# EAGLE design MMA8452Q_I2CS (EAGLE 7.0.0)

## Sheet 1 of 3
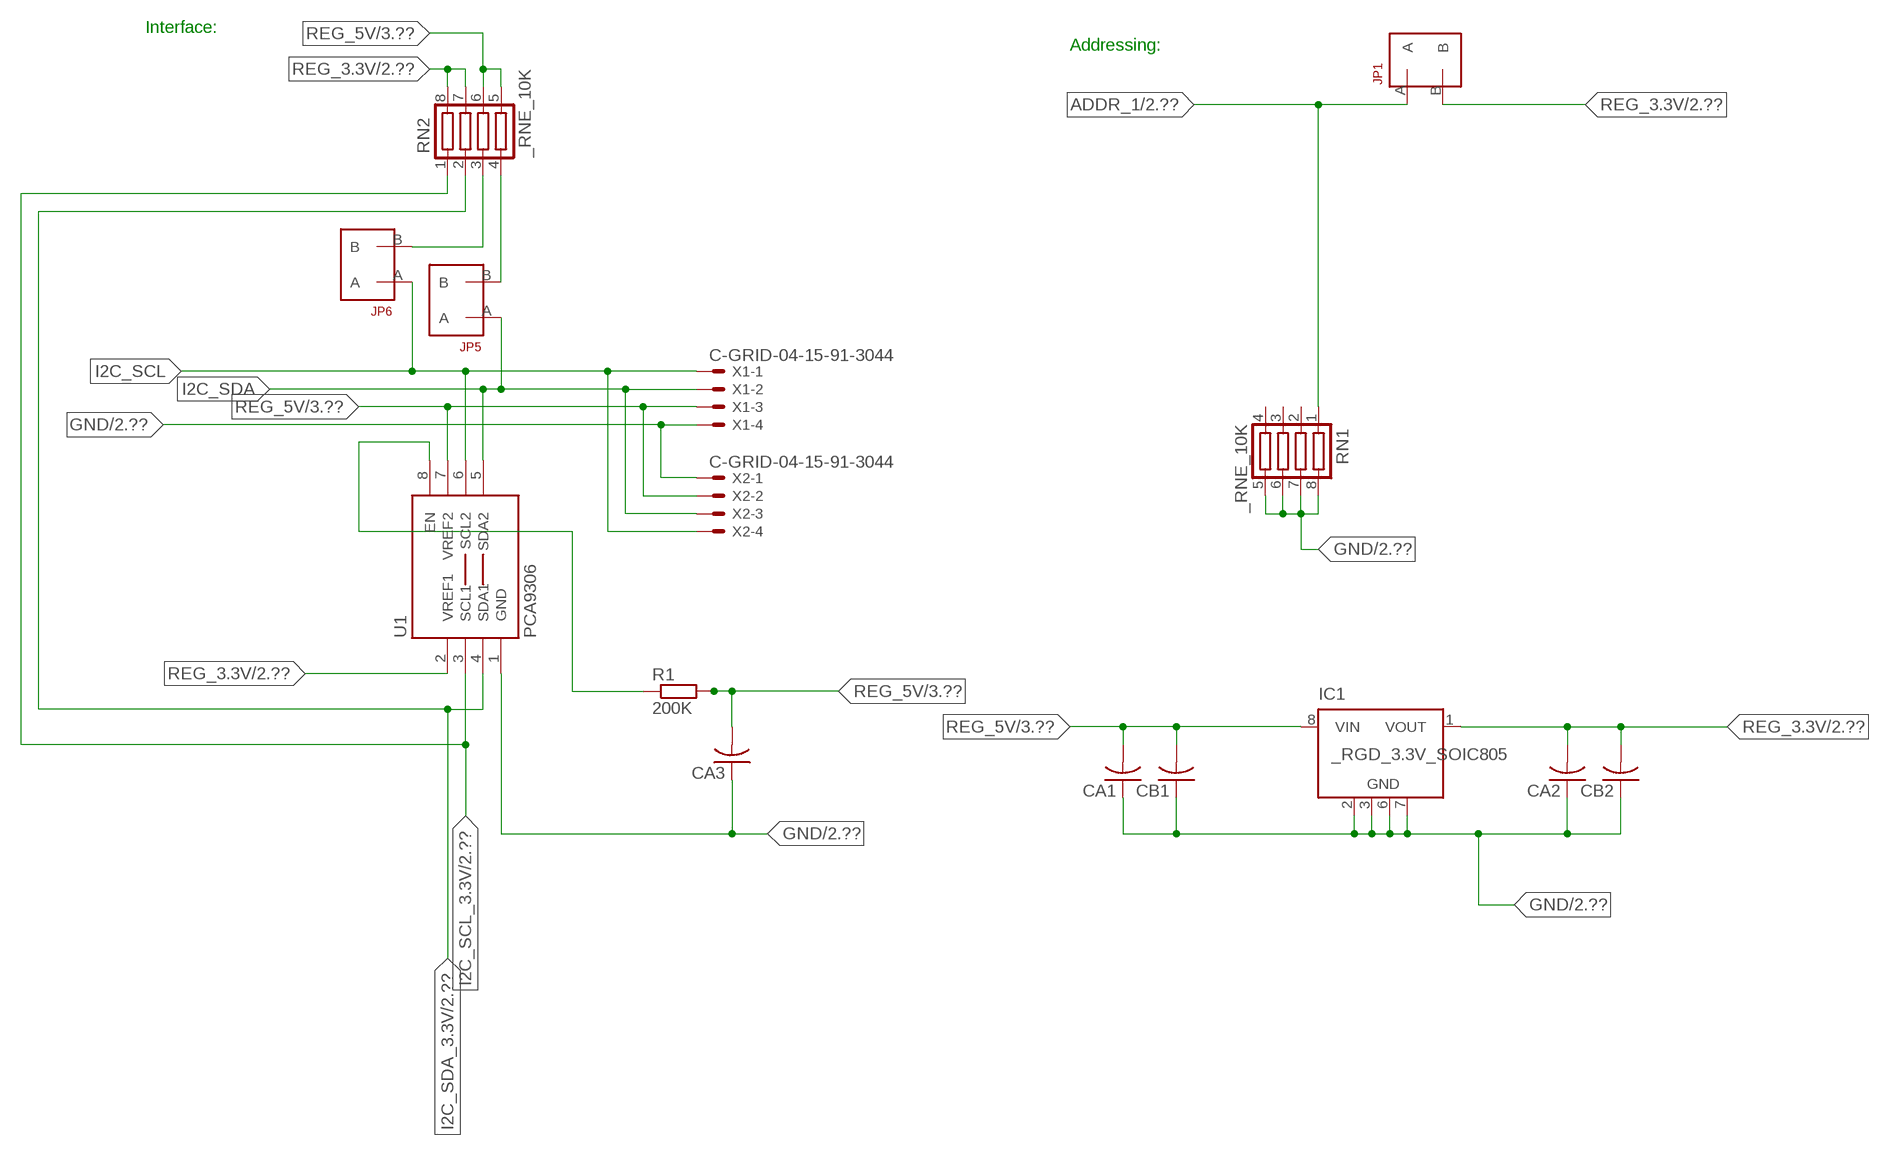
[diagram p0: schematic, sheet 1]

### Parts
CA1  CC1206KRX7R9BB104  [.1UF]
CA2  CC1206KRX7R9BB104  [.1UF]
CA3  CC1206KRX7R9BB104  [.1UF]
CB1  TMK316F106ZL-TC1206K  [TMK316F106ZL-T]
CB2  TMK316F106ZL-TC1206K  [TMK316F106ZL-T]
IC1  _RGD_3.3V_SOIC805  [_RGC_3.3V_SOIC8]
JP1  JUMPER_1X2_2MM  [JUMPER_1X2_2MM]
JP5  JUMPER_1X2_2MM  [JUMPER_1X2_2MM]
JP6  JUMPER_1X2_2MM  [JUMPER_1X2_2MM]
R1  200K  RESISTOR_SMT-0603  [R603]
RN1  _RNE_10K  [RNE]
RN2  _RNE_10K  [RNE]
U1  PCA9306  PCA9306_NCD  [PSOP-8]
X1  C-GRID-04-15-91-3044  [15-91-04]
X2  C-GRID-04-15-91-3044  [15-91-04]

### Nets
ADDR_1: JP1.A RN1.1 ; also sheet 2
GND: CA1.1 CA2.1 CA3.1 CB1.1 CB2.1 IC1.2(GND) IC1.3(GND) IC1.6(GND) IC1.7(GND) RN1.5 RN1.6 RN1.7 RN1.8 U1.1(GND) X1.4 X2.1 ; also sheet 2,3
I2C_SCL: JP6.A U1.6(SCL2) X1.1 X2.4
I2C_SCL_3.3V: RN2.1 U1.3(SCL1) ; also sheet 2
I2C_SDA: JP5.A U1.5(SDA2) X1.2 X2.3
I2C_SDA_3.3V: RN2.2 U1.4(SDA1) ; also sheet 2
N$1: JP6.B RN2.3
N$2: JP5.B RN2.4
N$3: R1.1 U1.8(EN)
REG_3.3V: CA2.2 CB2.2 IC1.1(VOUT) JP1.B RN2.7 RN2.8 U1.2(VREF1) ; also sheet 2
REG_5V: CA1.2 CA3.2 CB1.2 IC1.8(VIN) R1.2 RN2.5 RN2.6 U1.7(VREF2) X1.3 X2.2 ; also sheet 3
Unconnected: IC1.4(NC) IC1.5(NC) RN1.2 RN1.3 RN1.4

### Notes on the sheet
- Interface:
- Addressing:

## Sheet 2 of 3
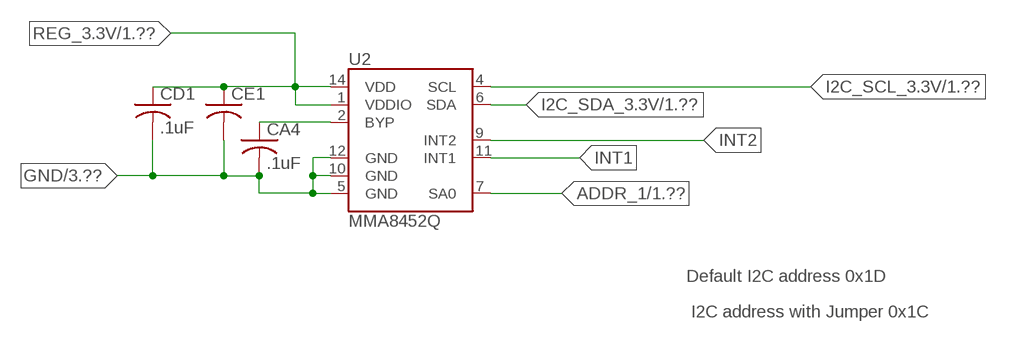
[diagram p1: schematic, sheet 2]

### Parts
CA4  .1uF  CC1206KRX7R9BB104  [.1UF]
CD1  .1uF  CC1206KRX7R9BB103C1206K  [CC1206KRX7R9BB103]
CE1  10uF  CC0603JRNPO8BN1020603  [CC0603JRNPO8BN102]
U2  MMA8452Q  [QFN-16_0.5MM]

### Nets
ADDR_1: U2.7(SA0) ; also sheet 1
GND: CA4.2 CD1.2 CE1.2 U2.5(GND) U2.10(GND) U2.12(GND) ; also sheet 1,3
I2C_SCL_3.3V: U2.4(SCL) ; also sheet 1
I2C_SDA_3.3V: U2.6(SDA) ; also sheet 1
INT1: U2.11(INT1)
INT2: U2.9(INT2)
N$6: CA4.1 U2.2(BYP)
REG_3.3V: CD1.1 CE1.1 U2.1(VDDIO) U2.14(VDD) ; also sheet 1

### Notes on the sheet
- Default I2C address 0x1D
- I2C address with Jumper 0x1C

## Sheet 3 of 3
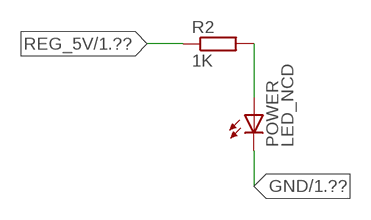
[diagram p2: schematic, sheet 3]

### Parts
POWER  LED_NCD  [CHIPLED_0603]
R2  1K  RESISTOR_SMT-0402  [R402]

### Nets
GND: POWER.C ; also sheet 1,2
N$4: POWER.A R2.2
REG_5V: R2.1 ; also sheet 1

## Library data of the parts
CA1-CA4 = NCD_ULTIMATE_LIBRARY:CC1206KRX7R9BB104: Capacitor CA .1uF 50V SMT C1206K CC1206KRX7R9BB104
CB1 CB2 = NCD_ULTIMATE_LIBRARY:TMK316F106ZL-T: Capacitor CB 10uF SMT 1206 TMK316F106ZL-T
CD1 = NCD_ULTIMATE_LIBRARY:CC1206KRX7R9BB103: Capacitor CD .01uF SMT CC1206KRX7R9BB103 1206
CE1 = NCD_ULTIMATE_LIBRARY:CC0603JRNPO8BN102: Capacitor CE 1uF SMT CC0603JRNPO8BN102 0603
IC1 = NCD_ULTIMATE_LIBRARY:_RGD_3.3V_SOIC8: Regulator Linear 3.3V Chip Positive VOLTAGE REGULATOR Digikey 497-1199-2-ND/L78L33ACD13TR
JP1 JP5 JP6 = NCD_ULTIMATE_CONNECTORS:JUMPER_1X2_2MM
POWER = NCD_ULTIMATE_LIBRARY:LED_NCD: LED Digikey 754-1132-2-ND/APT2012SRCPRV
R1 R2 = NCD_ULTIMATE_LIBRARY:RESISTOR_SMT: NCD Resistor
RN1 RN2 = NCD_ULTIMATE_LIBRARY:_RNE_10K: Resistor Array RNE SMT 10K x 4 Single Resistor Source: http://www.ctscorp.com/components/Datasheets/CTSChipArrayDs.pdf Digikey 742C083103JPTR-ND/742C083103JP; OC_FARNELL: unknown; OC_NEWARK: unknown
U1 = NCD_ULTIMATE_LIBRARY:PCA9306_NCD: NCD Bidirectional I2C level shifter. NOT compatible with all available part number pinout schemes- DOUBLE CHECK!!!; PROD_ID: IC-10023
U2 = NCD_ULTIMATE_bhaskar:MMA8452Q: MMA8452Q 3-Axis Digikey MMA8452QR1TR-ND/MMA8452QR1, 12/8-bit Digital Accelerometer Supply Voltage: 1.6-3.6V Range: +/- 2g, 4g, 8g Interface: I2C, 12-bit and 8-bit ODR: 1.56 Hz - 800 Hz Package: QFN-16 http://cache.freescale.com/files/sensors/doc/data_sheet/MMA8452Q.pdf; PROD_ID: IC-10769
X1 X2 = NCD_ULTIMATE_CONNECTORS:C-GRID-04: CONNECTOR 4-Pos I2C wire to board 2.54 mm (0.100") pitch header Digikey WM1342-ND/0015912045; OC_FARNELL: unknown; OC_NEWARK: unknown

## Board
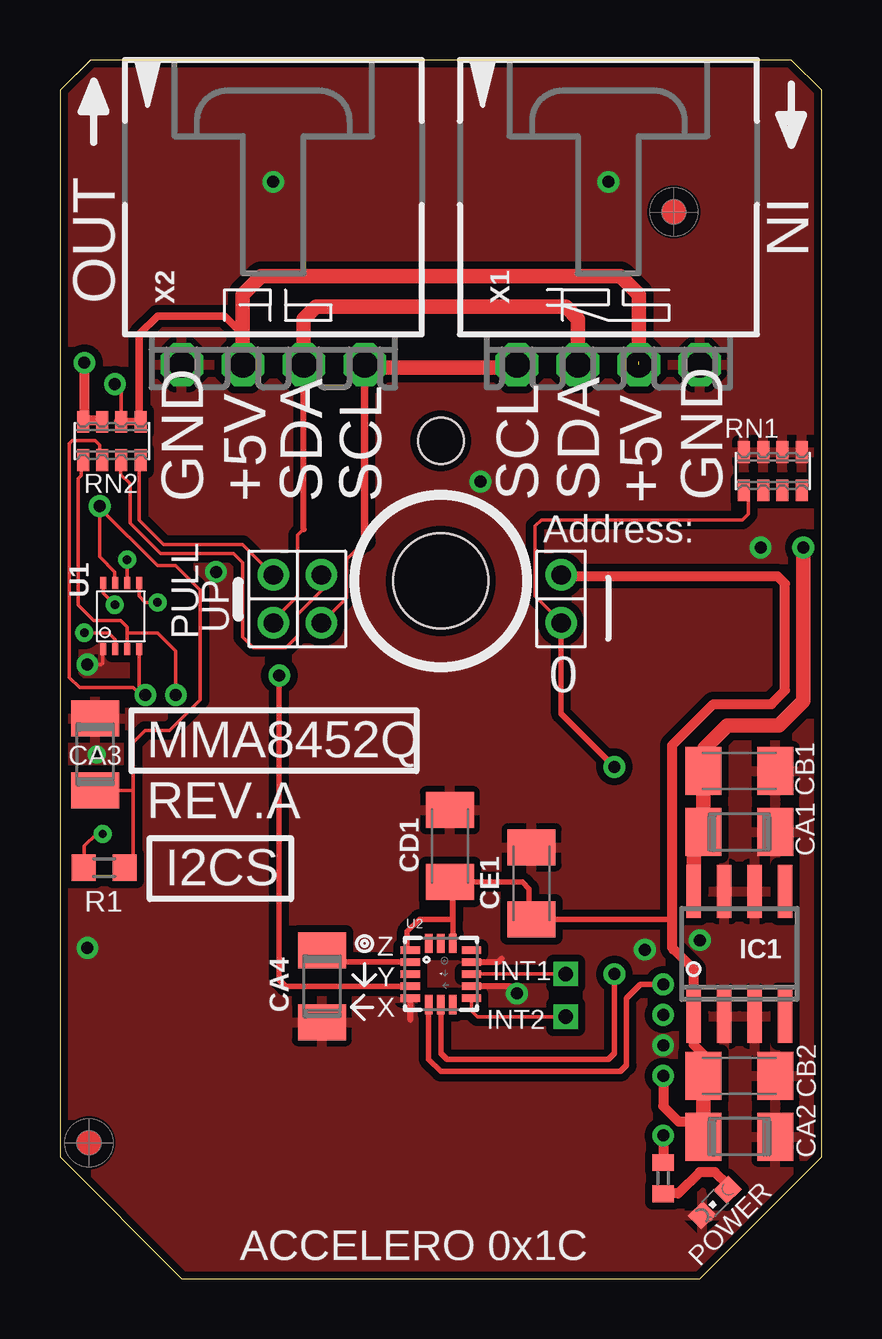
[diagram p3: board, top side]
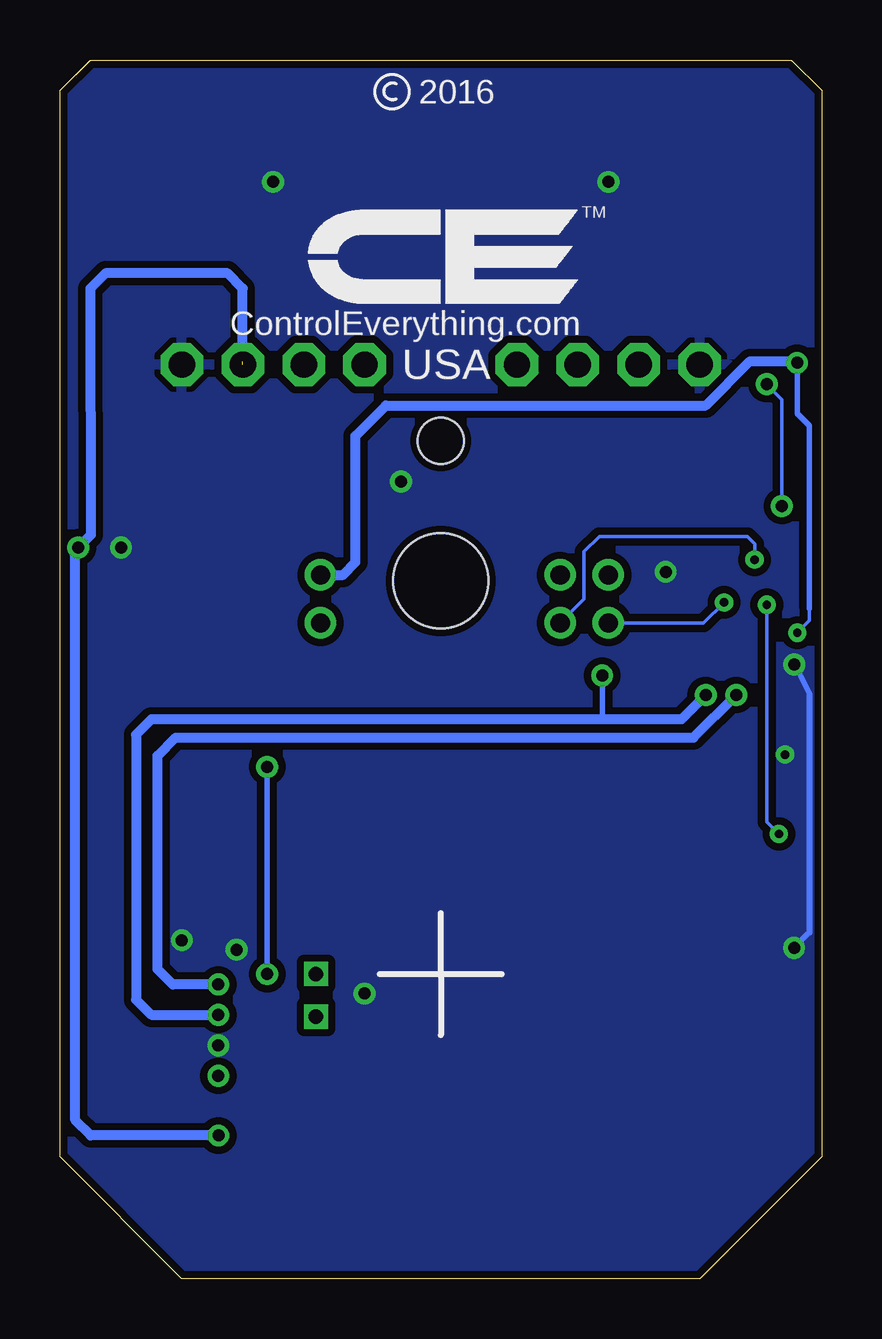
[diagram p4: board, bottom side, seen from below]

Size 31.75 x 50.8 mm. Coordinates in mm from the lower left corner, seen from the top.
Outline: 32 segments
Copper layers (1*16): Top 0.035mm / dielectric 1.5mm / Bottom 0.035mm
Design rules "default": minimum track width 5mil, minimum drill 24mil, track to track 5mil, track to pad 5mil, pad to pad 5mil, via to via 5mil, smd to smd 5mil, copper to edge 10mil, drill to drill 8mil, minimum pad ring 10mil, minimum via ring 8mil, stop-mask expansion 2mil, vias tented up to drill 0mil, thermal gap 10mil
Holes 3.96 mm at 15.88,29.08
Holes 1.91 mm at 15.88,34.93

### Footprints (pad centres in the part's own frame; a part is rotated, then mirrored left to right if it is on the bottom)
.1UF = smd 1.5 x 2: 1 -1.5,0; 2 1.5,0
TMK316F106ZL-T = smd 1.5 x 2: 1 -1.5,0; 2 1.5,0
CC1206KRX7R9BB103 = smd 1.5 x 2: 1 -1.5,0; 2 1.5,0
CC0603JRNPO8BN102 = smd 1.5 x 2: 1 -1.5,0; 2 1.5,0
_RGC_3.3V_SOIC8 = smd 0.6 x 2.2: 1 -1.905,-2.6; 2 -0.635,-2.6; 3 0.635,-2.6; 4 1.905,-2.6; 5 1.905,2.6; 6 0.635,2.6; 7 -0.635,2.6; 8 -1.905,2.6
JUMPER_1X2_2MM = drill 0.8: A 0,2; B 0,0
CHIPLED_0603 = smd 0.8 x 0.876: A 0,-0.75; C 0,0.75
R603 = smd 1 x 1.1: 1 -0.85,0; 2 0.85,0
R402 = smd 0.7 x 0.9: 1 -0.65,0; 2 0.65,0
RNE = smd 0.5 x 0.9: 1 -1.2,-0.8; 2 -0.4,-0.8; 3 0.4,-0.8; 4 1.2,-0.8; 5 1.2,0.8; 6 0.4,0.8; 7 -0.4,0.8; 8 -1.2,0.8
PSOP-8 = smd 0.25 x 0.5: 1 -0.73,-1.37; 2 -0.23,-1.37; 3 0.27,-1.37; 4 0.77,-1.37; 5 0.77,1.38; 6 0.27,1.38; 7 -0.23,1.38; 8 -0.73,1.38
QFN-16_0.5MM = smd 0.8 x 0.3: 1 -1.275,1; 2 -1.275,0.5; 3 -1.275,0; 4 -1.275,-0.5; 5 -1.275,-1; 9 1.275,-1; 10 1.275,-0.5; 11 1.275,0; 12 1.275,0.5; 13 1.275,1 | smd 0.3 x 0.8: 6 -0.5,-1.275; 7 0,-1.275; 8 0.5,-1.275; 14 0.5,1.275; 15 0,1.275; 16 -0.5,1.275
15-91-04 = drill 1.1 pad 1.778 octagon: 1 -3.81,-7.62; 2 -1.27,-7.62; 3 1.27,-7.62; 4 3.81,-7.62

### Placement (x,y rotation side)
CA1  28.32,18.62 180 top
CA2  28.32,5.92 180 top
CA3  1.46,21.86 270 top
CA4  10.92,12.19 270 top
CB1  28.32,21.16 180 top
CB2  28.32,8.46 180 top
CD1  16.26,18.03 90 top
CE1  19.66,16.48 90 top
IC1  28.32,13.54 0 top
JP1  20.89,29.34 180 top
JP5  8.89,29.34 180 top
JP6  10.9,29.34 180 top
POWER  27.3,3.18 135 top
R1  1.84,17.13 0 top
R2  25.15,4.19 270 top
RN1  29.72,33.66 0 top
RN2  2.16,34.93 0 top
U1  2.54,27.61 0 top
U2  15.88,12.7 0 top
U$5  [VISION_REF10]  1.21,5.66 90 top
U$28  [VISION_REF10]  25.59,44.46 90 top
X1  22.86,45.72 0 top
X2  8.89,45.72 0 top

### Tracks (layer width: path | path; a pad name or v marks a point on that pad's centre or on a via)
ADDR_1  (via drill 0.5)
  Top 0.152: JP1.A 20.89,27.37 19.81,28.45 19.81,31.37 20.07,31.62 28.45,31.62 28.7,31.88 28.7,32.78 RN1.1
  Top 0.229: U2.7 15.88,9.4 16.13,9.14 22.86,9.14 23.11,9.4 v23.11,12.7 | v23.11,21.34 20.89,23.56 JP1.A
  Bottom 0.229: v23.11,12.7 v23.11,21.34
GND  (via drill 0.35, 0.5)
  Top 0.152: CA3.1 1.52,23.42 1.52,23.62 | U1.1 1.78,26.21 1.78,25.65 1.73,25.6 v1.14,25.6
  Top 0.254: U2.12 18.28,13.2 18.41,13.34 | U2.5 14.6,10.8 14.61,10.8 | U2.10 18.74,12.2 v19.05,11.89
  Bottom 0.254: v1.14,25.6 1.02,25.4 0.51,24.38 0.51,14.43 v1.15,13.79
  other vias: 8.89,45.72 22.86,45.72 25.15,9.73 17.53,33.22 26.67,14.11 6.5,29.46 24.38,13.72 29.21,30.48 1.52,21.84
  pour Bottom (isolate 0.305): -0.64,5.08 -0.64,49.53 1.27,51.44 30.48,51.44 32.38,49.53 32.38,5.08 26.67,-0.63 5.08,-0.63
  pour Top (isolate 0.305): 4.45,-1.27 -1.27,4.45 -1.27,50.17 0.64,52.07 31.11,52.07 33.02,50.17 33.02,4.45 27.3,-1.27
I2C_SCL  (via drill 0.35)
  Top 0.152: 12.7,30.73 11.94,29.97 11.94,28.38 JP6.A | v2.79,29.97 2.81,29.96 U1.6
  Top 0.305: 12.7,30.73 X2.4
  Top 0.406: X2.4 12.7,37.97 | 19.05,37.97 X1.1
  Top 0.61: 12.7,37.97 19.05,37.97
  Bottom 0.152: JP6.A 9.91,28.33 9.91,30.3 9.27,30.94 3.1,30.94 2.79,30.63 v2.79,29.97
I2C_SCL_3.3V  (via drill 0.5)
  Top 0.152: RN2.1 0.89,34.07 0.89,33.48 0.77,33.35 0.77,28.08 1.41,27.43 2.54,27.43 2.81,27.17 2.81,26.92 | 2.81,26.92 U1.3 | v4.83,24.33 v4.83,24.34 4.83,26.16 4.06,26.92 2.81,26.92
  Top 0.229: U2.4 14.46,12.19 9.4,12.19 9.14,12.45 v9.14,25.15
  Bottom 0.229: v9.14,25.15 9.14,23.32
  Bottom 0.406: v4.83,24.33 5.84,23.32 9.14,23.32 27.94,23.32 28.58,22.68 28.58,11.63 27.94,11 v25.15,11
I2C_SDA  (via drill 0.35)
  Top 0.152: JP5.A 8.89,27.44 9.91,28.45 9.91,30.99 10.16,31.24 | U1.5 3.3,28.45 3.56,28.19 v4.06,28.19
  Top 0.254: 10.16,31.24 10.16,31.25 X2.3
  Top 0.61: X2.3 10.16,40.01 10.67,40.51 21.09,40.51 21.59,40.01 X1.2
  Bottom 0.152: v4.06,28.19 4.92,27.34 JP5.A
I2C_SDA_3.3V  (via drill 0.5)
  Top 0.152: RN2.2 1.65,34.14 1.65,34.75 1.46,34.94 0.51,34.94 0.38,34.81 0.38,26.37 0.38,26.36 0.38,25.07 0.81,24.64 3.05,24.64 3.35,24.33 v3.56,24.33 3.31,24.58 U1.4
  Top 0.229: U2.6 15.37,11.42 15.37,9.14 15.88,8.64 23.37,8.64 23.62,8.89 23.62,11.68 24.21,12.27 v25.15,12.27
  Bottom 0.406: v25.15,12.27 27.05,12.27 27.69,12.9 27.69,21.79 26.93,22.56 5.34,22.56 v3.56,24.33
INT1  (via drill 0.6)
  Top 0.152: U2.11 v21.08,12.7
INT2  (via drill 0.6)
  Top 0.152: 17.02,11.7 U2.9 17.15,11.17 17.4,10.92 v21.08,10.92
N$1
  Top 0.152: JP6.B 10.92,29.31 10.92,28.7 9.91,27.69 9.91,26.8 9.42,26.31 8.06,26.31 7.62,26.75 7.62,29.84 7.24,30.23 4.19,30.23 2.92,31.5 2.92,33.15 2.54,33.53 2.54,34.1 RN2.3
  Top 0.305: 2.54,34.02 RN2.3
N$2
  Top 0.152: JP5.B 7.62,30.61 4.32,30.61 3.3,31.62 3.3,34.07 RN2.4
  Top 0.305: 3.37,33.88 RN2.4
N$3  (via drill 0.35)
  Top 0.152: R1.1 1.02,17.16 1.02,18.03 1.52,18.54 v1.78,18.54 | 1.81,28.67 U1.8 1.81,28.57 v2.29,28.09
  Bottom 0.152: v1.78,18.54 2.29,19.05 v2.29,28.09
N$4
  Top 0.406: POWER.A 27.84,3.92 27.3,4.45 26.67,4.45 25.78,3.56 25.16,3.56 R2.2
N$6
  Top 0.229: CA4.1 11.7,13.2 U2.2
REG_3.3V  (via drill 0.35, 0.5)
  Top 0.152: v1.02,26.92 2.03,26.92 2.31,26.65 U1.2
  Top 0.229: U2.14 16.38,14.1 16.38,14.99 14.99,14.99 14.48,14.48 14.48,13.71 U2.1 | 25.53,14.99 CE1.1 19.56,15.09 19.56,16.26 19.28,16.53 CD1.1
  Top 0.254: 16.38,14.99 16.38,16.41 CD1.1
  Top 0.305: 25.53,13.69 25.53,13.79
  Top 0.406: CB2.2 26.82,9.35 26.42,9.75 26.42,10.36 | v25.15,8.46 25.15,7.19 25.78,6.55 26.82,6.55 | IC1.1 26.42,12.9 25.53,13.79 25.53,14.99 25.53,22.24 27.24,23.95 29.66,23.95 30.23,24.52 30.23,28.97 29.91,29.29 20.95,29.29 JP1.B | 26.52,5.62 CA2.2 | v1.02,38.18 1.02,35.78 | 1.02,35.78 RN2.8 | 1.02,35.78 1.71,35.78 RN2.7
  Top 0.61: CB2.2 26.82,6.55 CA2.2 | 26.42,10.36 IC1.1
  Bottom 0.152: 0.51,27.94 0.51,27.43 v1.02,26.92
  Bottom 0.229: 0.51,27.94 0.51,35.56 1.02,36.07 v1.02,38.18
  Bottom 0.406: v1.02,38.18 1.08,38.24 2.99,38.24 4.83,36.4 18.16,36.4 19.43,35.13 19.43,29.87 19.94,29.34 JP1.B
REG_5V  (via drill 0.5)  (1 unrouted)
  Top 0.152: RN2.6 2.56,37.01 v2.29,37.29 | R1.2 3.05,17.49 3.05,20.36 | 3.05,20.36 3.05,22.35 3.56,22.86 4.57,22.86 5.84,24.13 5.84,28.7 4.83,29.72 4.06,29.72 1.65,32.13 v1.65,32.21 1.65,30.1 2.29,29.46 2.29,29.01 U1.7 | CA3.2 3.05,20.36
  Top 0.305: 7.62,39.37 7.5,39.37 | 2.42,35.74 RN2.6 RN2.5 3.31,35.8 3.31,39.37 4.07,40.13 6.86,40.13 7.62,39.37 | X2.2 7.62,39.37
  Top 0.406: v25.15,5.97 R2.1
  Top 0.61: X2.2 7.62,41.02 8.38,41.78 23.37,41.78 24.13,41.02 X1.3 | IC1.8 26.42,18.21 CA1.2 CB1.2 26.86,21.2 26.86,22.11 27.82,23.06 29.98,23.06 30.99,24.08 v30.99,30.48
  Bottom 0.152: v1.65,32.21 1.65,36.65 v2.29,37.29
  Bottom 0.406: 24.13,38.23 24.13,41.28 24.77,41.91 29.85,41.91 30.48,41.27 30.47,31 v30.99,30.48 31.11,30.36 31.11,6.6 30.48,5.97 v25.15,5.97

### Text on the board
tPlace: Z | Y | X | ACCELERO 0x1C
tNames: IN | OUT | GND | +5V | SDA | SCL | SCL | SDA | +5V | GND | Address: | PULL | UP | 0 | MMA8452Q | REV.A | I2CS | INT1 | INT2
bNames: 2016 | TM | ControlEverything.com | USA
